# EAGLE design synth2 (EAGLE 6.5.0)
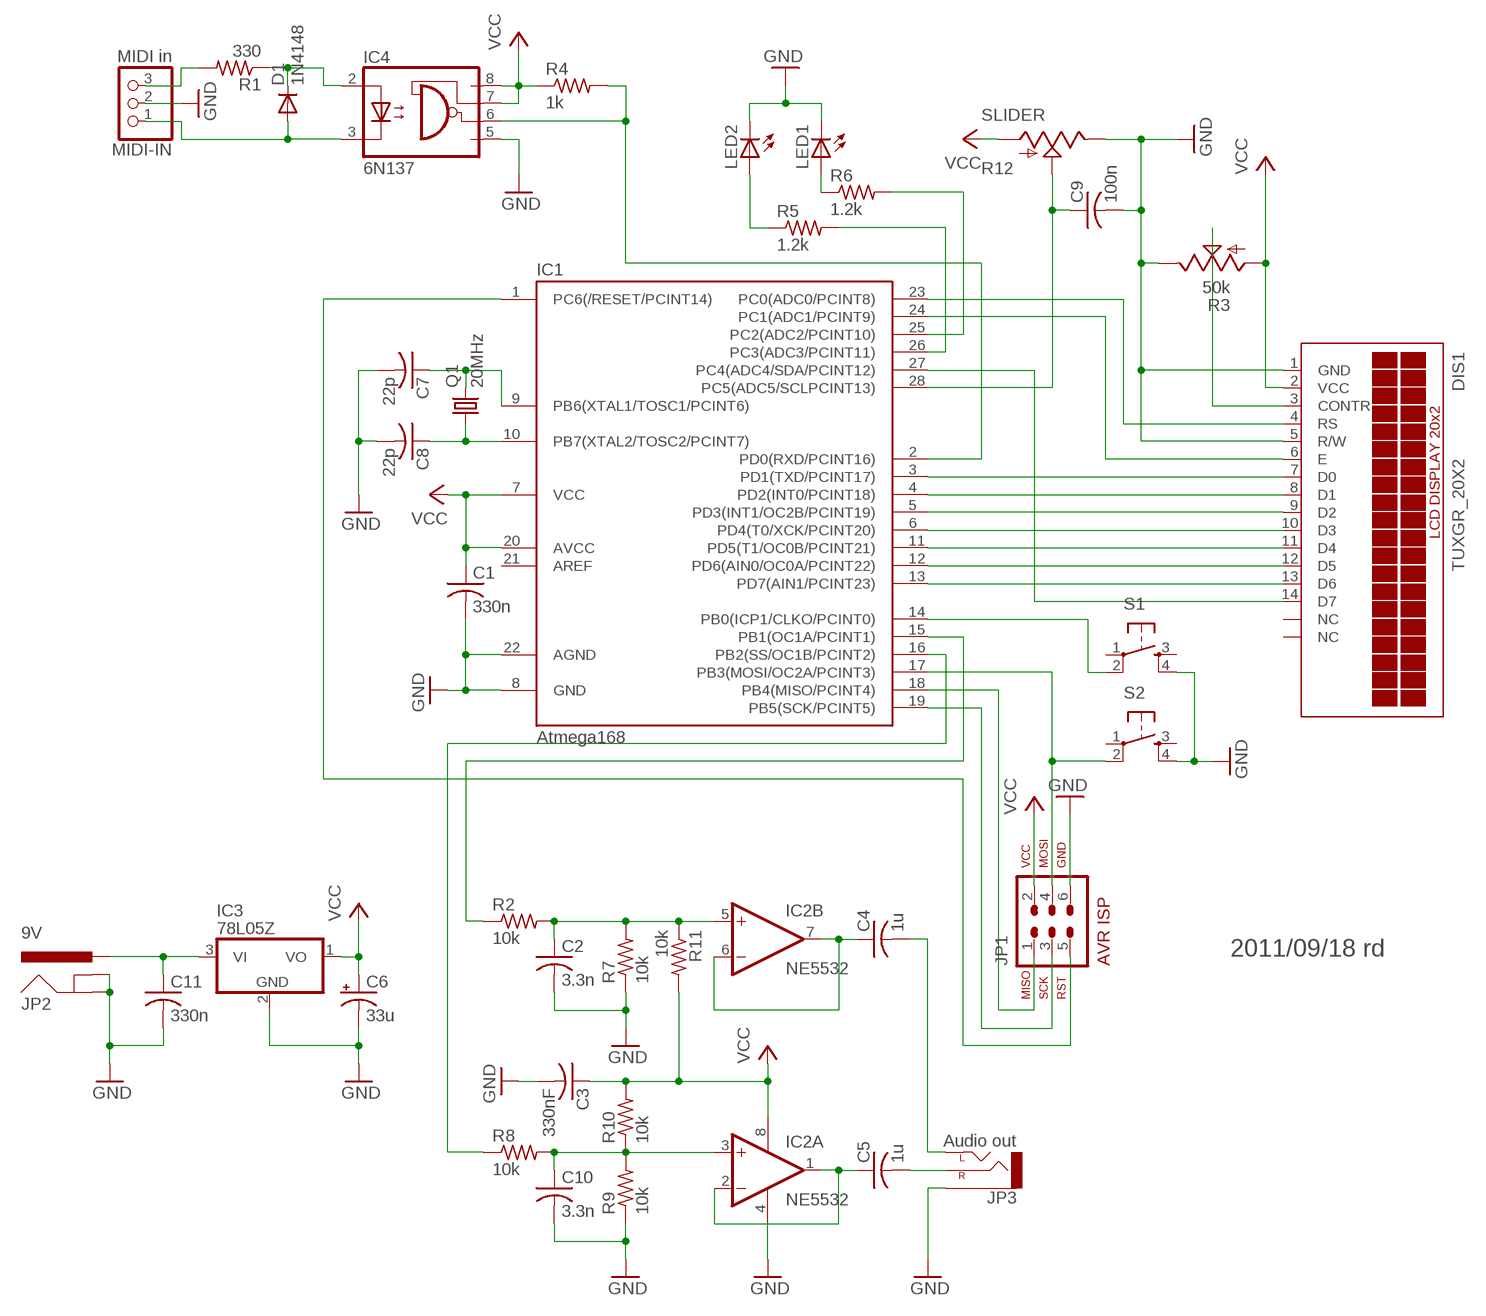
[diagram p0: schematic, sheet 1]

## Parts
C1  330n  C-USC0805  [C0805]
C2  3.3n  C-USC0805  [C0805]
C3  330nF  C-USC0805  [C0805]
C4  1u  C-USC0805  [C0805]
C5  1u  C-USC0805  [C0805]
C6  33u  CPOL-USCT7343  [CT7343]
C7  22p  C-USC0805  [C0805]
C8  22p  C-USC0805  [C0805]
C9  100n  C-USC0805  [C0805]
C10  3.3n  C-USC0805  [C0805]
C11  330n  C-USC0805  [C0805]
D1  1N4148  DIODE-SOD80C  [SOD80C]
DIS1  TUXGR_20X2  [TUXGR_20X2]
IC1  Atmega168  MEGA48/88/168-PU  [DIL28-3]
IC2  NE5532  TLC27L2ACP  [DIL08]
IC3  78L05Z  [TO92]
IC4  6N137  [DIL08]
JP1  AVR-ISP-6VERT  [AVR-ISP-6]
JP2  9V  POWER_JACKPTH  [POWER_JACK_PTH]
JP3  Audio out  AUDIO-JACKPTH  [AUDIO-JACK]
LED1  LED5MM  [LED5MM]
LED2  LED5MM  [LED5MM]
MIDI-IN  MIDI in  PINHD-1X3M  [1X03M]
Q1  20MHz  CRYSTALHC49U70  [HC49U70]
R1  330  R-US_R0805  [R0805]
R2  10k  R-US_R0805  [R0805]
R3  50k  TRIM_US-CA6V  [CA6V]
R4  1k  R-US_R0805  [R0805]
R5  1.2k  R-US_R0805  [R0805]
R6  1.2k  R-US_R0805  [R0805]
R7  10k  R-US_R0805  [R0805]
R8  10k  R-US_R0805  [R0805]
R9  10k  R-US_R0805  [R0805]
R10  10k  R-US_R0805  [R0805]
R11  10k  R-US_R0805  [R0805]
R12  SLIDER  [SLIDER]
S1  TAC_SWITCHPTH  [TACTILE-PTH]
S2  TAC_SWITCHPTH  [TACTILE-PTH]

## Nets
GND [Power]: C1.2 C2.2 C3.2 C6.- C7.2 C8.2 C9.2 C10.2 C11.2 DIS1.1(GND) DIS1.5(R/W) IC1.8(GND) IC1.22(AGND) IC2.4(C:GND) IC3.2(GND) IC4.5(GND) JP1.6 JP2.GND JP2.GNDBREAK JP3.SLEEVE LED1.K(C) LED2.K(C) MIDI-IN.2 R3.E R7.1 R9.1 R12.1(E) S1.4 S2.4
N$1: IC1.1(PC6(/RESET/PCINT14)) JP1.5
N$2: DIS1.4(RS) IC1.23(PC0(ADC0/PCINT8))
N$3: DIS1.6(E) IC1.24(PC1(ADC1/PCINT9))
N$4: D1.C IC4.2(A) R1.1
N$5: D1.A IC4.3(C) MIDI-IN.1
N$6: MIDI-IN.3 R1.2
N$7: DIS1.7(D0) IC1.3(PD1(TXD/PCINT17))
N$8: IC1.17(PB3(MOSI/OC2A/PCINT3)) JP1.4 S2.2
N$9: IC1.18(PB4(MISO/PCINT4)) JP1.1
N$10: IC1.19(PB5(SCK/PCINT5)) JP1.3
N$11: C2.1 IC2.5(B:+IN) R2.2 R7.2 R11.1
N$12 [Power]: DIS1.3(CONTR) R3.S
N$13: C4.1 IC2.6(B:-IN) IC2.7(B:OUT)
N$14: IC1.16(PB2(SS/OC1B/PCINT2)) R8.1
N$15: C4.2 JP3.TIP(LEFT)
N$16: C10.1 IC2.3(A:+IN) R8.2 R9.2 R10.1
N$17: C8.1 IC1.10(PB7(XTAL2/TOSC2/PCINT7)) Q1.1
N$18: C7.1 IC1.9(PB6(XTAL1/TOSC1/PCINT6)) Q1.2
N$19: IC1.15(PB1(OC1A/PCINT1)) R2.1
N$20: C9.1 IC1.28(PC5(ADC5/SCLPCINT13)) R12.2A(S)
N$21: IC1.14(PB0(ICP1/CLKO/PCINT0)) S1.2
N$22: DIS1.11(D4) IC1.11(PD5(T1/OC0B/PCINT21))
N$23: DIS1.8(D1) IC1.4(PD2(INT0/PCINT18))
N$24: DIS1.9(D2) IC1.5(PD3(INT1/OC2B/PCINT19))
N$25: DIS1.10(D3) IC1.6(PD4(T0/XCK/PCINT20))
N$26: DIS1.12(D5) IC1.12(PD6(AIN0/OC0A/PCINT22))
N$27: DIS1.13(D6) IC1.13(PD7(AIN1/PCINT23))
N$28: IC1.2(PD0(RXD/PCINT16)) IC4.6(VO) R4.2
N$29: IC1.25(PC2(ADC2/PCINT10)) R6.2
N$30: LED2.A R5.1
N$31: LED1.A R6.1
N$32: IC1.26(PC3(ADC3/PCINT11)) R5.2
N$33: DIS1.14(D7) IC1.27(PC4(ADC4/SDA/PCINT12))
N$35: C5.1 IC2.1(A:OUT) IC2.2(A:-IN)
N$36: C5.2 JP3.RING(RIGHT)
N$37: C11.1 IC3.3(VI) JP2.PWR
VCC [Power]: C1.1 C3.1 C6.+ DIS1.2(VCC) IC1.7(VCC) IC1.20(AVCC) IC2.8(C:VDD) IC3.1(VO) IC4.7(VE) IC4.8(VCC) JP1.2 R3.A R4.1 R10.2 R11.2 R12.3(A)
Unconnected: IC1.21(AREF) S1.1 S1.3 S2.1 S2.3

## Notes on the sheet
- 2011/09/18 rd

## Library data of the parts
C1-C5 C7-C11 = rcl:C-US: CAPACITOR, American symbol
C6 = rcl:CPOL-US: POLARIZED CAPACITOR, American symbol
D1 = diode:DIODE-: DIODE
DIS1 = display-lcd:TUXGR_20X2: Tuxgraphics LCD display 20x2 characters reflective, without background light Source: tuxgr_20x2.pdf; OC_FARNELL: unknown; OC_NEWARK: unknown
IC1 = avr-7:MEGA48/88/168-PU
IC2 = linear:TLC27L*: LinCMOS(TM) PRECISION DUAL OPERATIONAL AMPLIFIERS Source: http://focus.ti.com/lit/ds/symlink/tlc27l2.pdf
IC3 = linear:78*: Positive VOLTAGE REGULATOR Source: http://cache.national.com/ds/LM/LM78L05.pdf http://www.fairchildsemi.com/ds/LM/LM7805.pdf
IC4 = optocoupler:6N137: MOTOROLA OPTO COUPLER; MPN: 6N137; OC_FARNELL: 1328376; OC_NEWARK: 52M1895
JP1 = avr-7:AVR-ISP-6: AVR ISP-6 Serial Programming Header
JP2 = SparkFun-Connectors:POWER_JACK: Power Jack This is the standard 5.5mm barrel jack for power. The PTH is the most common, proven, reliable, footprint. The Slot footprint only works if the mill layer is transmitted to the PCB fab house so be warned. Mating wall wart : TOL-00298 (and others); PROD_ID: CONN-08197
JP3 = SparkFun:AUDIO-JACK: 3.5mm Audio Jack Simple 3.5mm common PCB mount audio jack. SKU: PRT-08032
LED1 LED2 = led:LED: LED
MIDI-IN = pinhead:PINHD-1X3: PIN HEADER
Q1 = crystal:CRYSTAL: CRYSTAL; OC_FARNELL: unknown; OC_NEWARK: unknown
R1 R2 R4-R11 = rcl:R-US_: RESISTOR, American symbol
R3 = pot:TRIM_US-: POTENTIOMETER
R12 = SparkFun:SLIDER
S1 S2 = SparkFun:TAC_SWITCH: Momentary Switch Button commonly used for reset or general input. Spark Fun Electronics SKU : COM-00097

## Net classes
0 default: width 0.254 mm
1 Power: width 0.508 mm

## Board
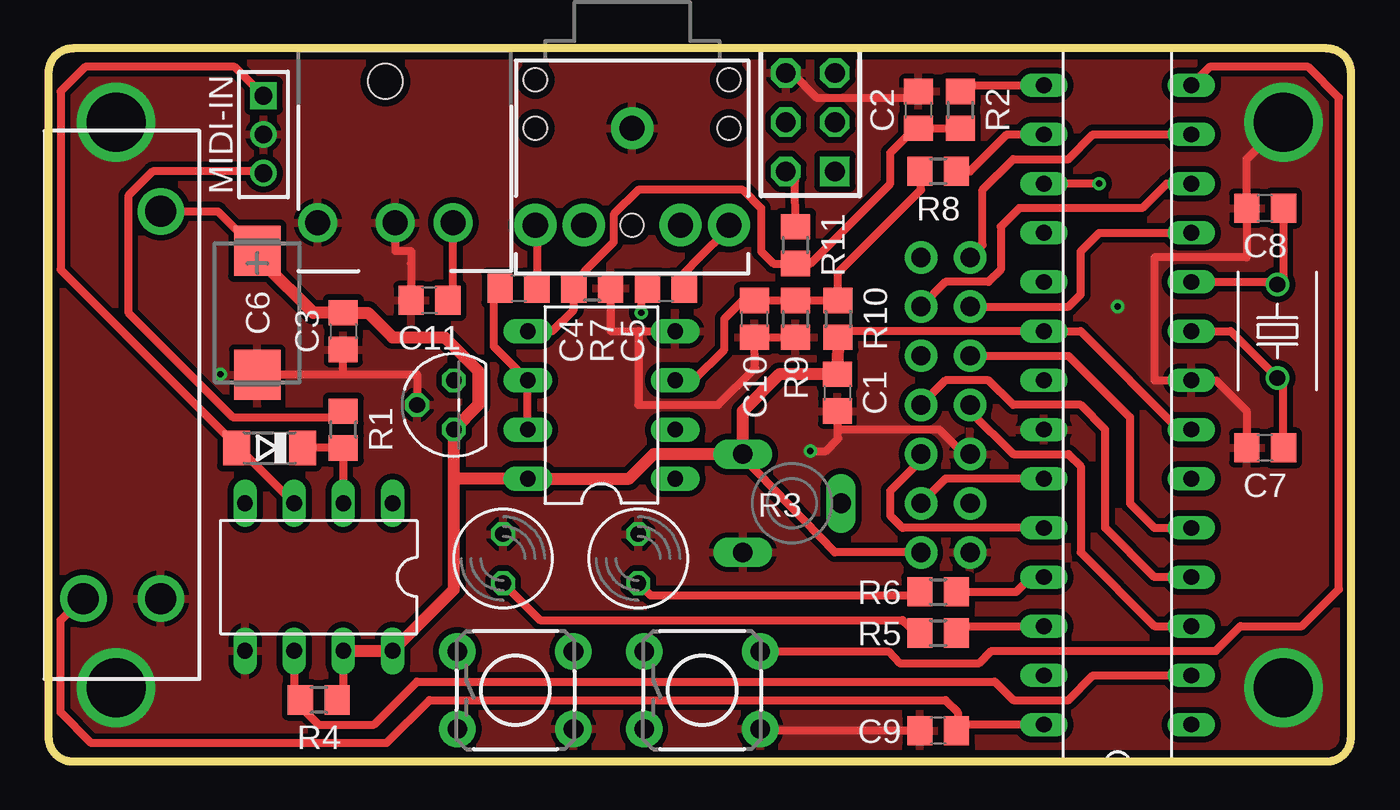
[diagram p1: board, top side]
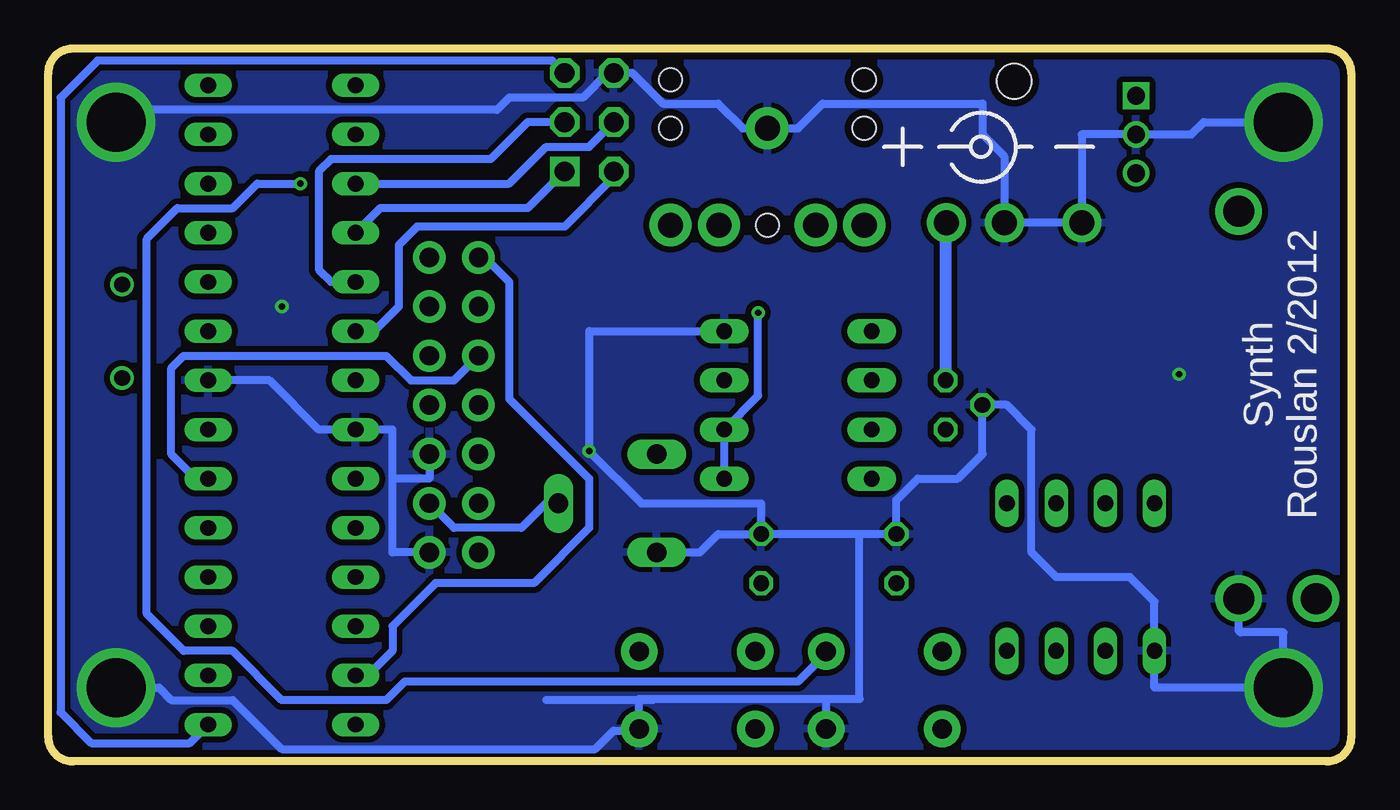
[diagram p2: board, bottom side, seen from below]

Size 67.31 x 36.83 mm. Coordinates in mm from the lower left corner, seen from the top.
Outline: 1.27,0 66.04,0 arc90 67.31,1.27 67.31,35.56 arc90 66.04,36.83 1.27,36.83 arc90 0,35.56 0,1.27 arc90 1.27,0
Copper layers (1*16): Top 0.0356mm / dielectric 1.5011mm / Bottom 0.0356mm
Design rules "LaenPCBOrder *": minimum track width 6mil, minimum drill 13mil, track to track 6mil, track to pad 6mil, pad to pad 6mil, via to via 6mil, smd to smd 6mil, copper to edge 15mil, drill to drill 6mil, minimum pad ring 7mil, minimum via ring 7mil, stop-mask expansion 3mil, vias tented up to drill 15mil, thermal gap 10mil

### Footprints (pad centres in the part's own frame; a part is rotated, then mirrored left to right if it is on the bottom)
C0805 = smd 1.3 x 1.5: 1 -0.95,0; 2 0.95,0
CT7343 = smd 2.6 x 2.4: + -3.2,0; - 3.2,0
SOD80C = smd 1.4 x 1.8: A 1.7,0; C -1.7,0
TUXGR_20X2 = drill 1 pad 1.676: 1 1.27,-7.62; 2 -1.27,-7.62; 3 1.27,-5.08; 4 -1.27,-5.08; 5 1.27,-2.54; 6 -1.27,-2.54; 7 1.27,0; 8 -1.27,0; 9 1.27,2.54; 10 -1.27,2.54; 11 1.27,5.08; 12 -1.27,5.08; 13 1.27,7.62; 14 -1.27,7.62
DIL28-3 = drill 0.813 long: 1 -16.51,-3.81; 2 -13.97,-3.81; 3 -11.43,-3.81; 4 -8.89,-3.81; 5 -6.35,-3.81; 6 -3.81,-3.81; 7 -1.27,-3.81; 8 1.27,-3.81; 9 3.81,-3.81; 10 6.35,-3.81; 11 8.89,-3.81; 12 11.43,-3.81; 13 13.97,-3.81; 14 16.51,-3.81; 15 16.51,3.81; 16 13.97,3.81; 17 11.43,3.81; 18 8.89,3.81; 19 6.35,3.81; 20 3.81,3.81; 21 1.27,3.81; 22 -1.27,3.81; 23 -3.81,3.81; 24 -6.35,3.81; 25 -8.89,3.81; 26 -11.43,3.81; 27 -13.97,3.81; 28 -16.51,3.81
DIL08 = drill 0.813 pad 1.27 long: 1 -3.81,-3.81; 2 -1.27,-3.81; 3 1.27,-3.81; 4 3.81,-3.81; 5 3.81,3.81; 6 1.27,3.81; 7 -1.27,3.81; 8 -3.81,3.81
TO92 = drill 0.813 octagon: 1 -1.27,0; 2 0,1.905; 3 1.27,0
DIL08' = drill 0.813 long: 1 -3.81,-3.81; 2 -1.27,-3.81; 3 1.27,-3.81; 4 3.81,-3.81; 5 3.81,3.81; 6 1.27,3.81; 7 -1.27,3.81; 8 -3.81,3.81
AVR-ISP-6 = drill 1.016 square: 1 -2.54,-1.27 | drill 1.016 octagon: 2 -2.54,1.27; 3 0,-1.27; 4 0,1.27; 5 2.54,-1.27; 6 2.54,1.27
POWER_JACK_PTH = drill 1.3 pad 2: GND 4.5,9; GNDBREAK 0.5,9; PWR -2.5,9 | hole 1.8: 1,1.7
AUDIO-JACK = drill 1.3 pad 2.184: RING 5,5; RSH 5,2.5; SLEEVE 0,0; TIP 5,-5; TSH 5,-2.5 | hole 1.2: 0,5; -2.5,5; -2.5,-5; 0,-5; 5,0
LED5MM = drill 0.813 octagon: A -1.27,0; K 1.27,0
1X03M = drill 0.914 square: 1 -2,0 | drill 0.914: 2 0,0; 3 2,0
HC49U70 = drill 0.813: 1 -2.413,0; 2 2.413,0
R0805 = smd 1.3 x 1.5: 1 -0.95,0; 2 0.95,0
CA6V = drill 1.016 long: A -2.54,-2.54; E 2.54,-2.54; S 0,2.54
SLIDER = drill 1.6 pad 2: 1 10,2; 2A 10,-2; 3 -10,2
TACTILE-PTH = drill 1.016 pad 1.88: 1 -3,2; 2 3,2; 3 -3,-2; 4 3,-2

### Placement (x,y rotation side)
C1  40.77,19.05 270 top
C2  44.96,33.65 90 top
C3  15.24,22.23 270 top
C4  24.29,24.45 0 top
C5  31.91,24.45 0 top
C6  10.79,23.18 270 top
C7  62.87,16.19 180 top
C8  62.87,28.57 180 top
C9  45.97,1.59 180 top
C10  36.48,22.86 270 top
C11  19.68,23.81 180 top
D1  11.43,16.19 180 top
DIS1  46.35,18.41 0 top
IC1  55.24,18.41 90 top
IC2  28.57,18.41 90 top
IC3  20.96,18.41 90 top
IC4  6N137  [DIL08']  13.97,9.53 180 top
JP1  39.37,33.02 90 top
JP2  18.41,36.83 180 top
JP3  30.16,32.7 270 top
LED1  30.48,10.48 90 top
LED2  23.5,10.48 90 top
MIDI-IN  11.11,32.38 270 top
Q1  63.5,22.23 270 top
R1  15.24,17.14 90 top
R2  47.12,33.65 270 top
R3  38.42,13.33 270 top
R4  13.97,3.17 180 top
R5  45.97,6.64 0 top
R6  45.97,8.76 0 top
R7  28.1,24.45 180 top
R8  45.97,30.48 180 top
R9  38.61,22.86 90 top
R10  40.8,22.86 270 top
R11  38.61,26.67 90 top
R12  3.81,18.41 270 top
S1  33.78,3.68 0 top
S2  24.13,3.68 0 top

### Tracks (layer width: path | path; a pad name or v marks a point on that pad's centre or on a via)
GND  (via drill 0.33, 3.05)
  Top 0.406: C7.2 61.91,18.09 60.32,19.69 IC1.8 57.15,19.69 57.15,26.03 61.91,26.03 C8.2 61.91,31.12 v63.82,33.02 | DIS1.5 47.31,15.87 46.04,17.14 40.8,17.14 | 40.8,17.14 C1.2 | R9.1 C10.2 36.51,20.32 34.61,18.41 30.48,18.41 30.48,22.23 | 30.48,22.23 29.05,22.23 R7.1 | 30.48,22.23 IC2.4 | C9.2 37.2,1.59 S1.4 | C6.- 10.82,20 15.24,20 | 15.24,20 C3.2 | 15.24,20 19.05,20 IC3.2 | JP1.6 38.42,35.56 39.69,34.29 44.77,34.29 C2.2 | v39.37,16.03 40.16,16.03 40.8,16.67 40.8,17.14 | JP2.GNDBREAK 17.91,26.38 18.73,26.38 18.73,25.72 C11.2
  Bottom 0.406: v3.49,33.02 7.62,33.02 8.26,32.38 MIDI-IN.2 13.92,32.38 JP2.GND JP2.GNDBREAK 17.91,31.25 19.05,32.38 19.05,33.97 27.3,33.97 28.57,32.7 JP3.SLEEVE 31.43,32.7 32.7,33.97 35.56,33.97 37.15,35.56 JP1.6 38.42,35.56 39.69,34.29 43.5,34.29 44.13,33.65 63.18,33.65 v63.82,33.02 | 25.4,11.75 LED2.K 23.5,13.49 22.38,14.6 20.32,14.6 19.05,15.87 IC3.2 17.78,18.41 16.51,17.14 16.51,10.79 15.24,9.53 11.43,9.53 10.16,8.26 IC4.5 10.16,3.81 v3.49,3.81 3.49,6.67 5.71,6.67 5.81,6.76 R12.1 | 25.4,11.75 LED1.K | 25.4,11.75 25.4,3.22 27.13,3.22 | 27.13,3.22 36.81,3.22 | 36.81,3.22 S1.4 36.88,1.59 38.1,1.59 39.05,0.63 55.24,0.63 57.78,3.17 60.96,3.17 61.59,3.81 v63.82,3.81 | 27.13,3.22 S2.4 | 36.81,3.22 36.07,3.17 41.59,3.17 | 49.53,14.6 47.62,14.6 DIS1.5 | 49.53,14.6 49.53,17.14 IC1.22 53.34,17.14 55.88,19.69 IC1.8 | DIS1.1 49.53,10.79 49.53,14.6 | R3.E 33.65,10.79 32.7,11.75 LED1.K | IC2.4 39.37,22.23 v39.37,16.03 36.67,13.33 30.48,13.33 LED1.K
  other vias: 8.89,20 8.89,20 55.24,23.49
  pour Bottom (isolate 0.305): -1.27,37.46 -1.27,-0.64 68.58,-0.64 68.58,37.46
  pour Top (isolate 0.305): -2.54,38.73 -2.54,-1.91 69.85,-1.91 69.85,38.73
N$1
  Bottom 0.406: JP1.5 41.27,36.2 64.77,36.2 66.67,34.29 66.67,2.54 65.09,0.95 60.01,0.95 IC1.1
N$2
  Top 0.406: IC1.23 46.35,14.6 DIS1.4
N$3
  Top 0.406: IC1.24 44.13,12.06 43.5,12.7 43.5,13.97 45.08,15.56 DIS1.6
N$4
  Top 0.406: IC4.2 R1.1 D1.C
N$5
  Top 0.406: IC4.3 9.84,16.19 D1.A 9.73,16.3 0.64,25.4 0.64,34.61 1.9,35.88 9.62,35.88 MIDI-IN.1
N$6
  Top 0.406: MIDI-IN.3 11.02,30.48 5.4,30.48 4.13,29.21 4.13,23.18 9.53,17.78 14.93,17.78 R1.2
N$7
  Top 0.406: DIS1.7 47.62,18.1 49.85,15.87 52.7,15.87 53.34,15.24 53.34,10.79 57.15,6.98 IC1.3
N$8  (via drill 0.33)
  Top 0.406: v54.29,29.84 IC1.17
  Bottom 0.406: IC1.17 43.5,29.84 41.59,31.75 39.37,31.75 JP1.4 | S2.2 27.13,5.57 28.57,4.13 48.89,4.13 49.85,3.17 55.24,3.17 57.78,5.71 60.32,5.71 62.23,7.62 62.23,26.99 60.64,28.57 57.78,28.57 56.51,29.84 v54.29,29.84
N$9
  Bottom 0.406: JP1.1 42.54,28.57 50.16,28.57 IC1.18
N$10
  Bottom 0.406: JP1.3 42.54,33.02 44.45,31.11 52.7,31.11 53.34,30.48 53.34,25.4 52.7,24.77 IC1.19
N$11
  Top 0.406: IC2.5 26.04,22.23 27.15,23.34 R7.2 27.78,25.4 29.21,26.83 29.21,28.26 30.48,29.53 35.88,29.53 36.83,28.57 36.83,26.35 37.46,25.72 38.41,25.72 R11.1 39.37,25.72 43.5,29.84 43.5,31.43 44.77,32.7 C2.1 R2.2
N$12
  Bottom 0.406: DIS1.3 46.35,12.06 42.86,12.06 41.59,13.33 R3.S
N$13
  Top 0.406: IC2.7 IC2.6 23.02,21.43 23.02,23.02 23.02,24.13 C4.1
N$14
  Top 0.406: R8.1 47.62,30.48 49.53,32.38 IC1.16
N$15
  Top 0.406: JP3.TIP 25.24,27.47 C4.2
N$16
  Top 0.406: IC2.3 33.34,19.69 34.92,21.27 34.92,22.86 35.88,23.81 36.51,23.81 C10.1 R9.2 R10.1 40.8,25.24 45.08,29.53 45.08,30.48 R8.2
  Bottom 0.406: IC2.3 33.34,19.69
N$17
  Top 0.406: C8.1 63.81,24.95 Q1.1 63.37,24.77 IC1.10
N$18
  Top 0.406: C7.1 63.81,19.5 Q1.2 61.09,22.23 IC1.9
N$19
  Top 0.406: R2.1 47.62,34.92 IC1.15
N$20
  Top 0.406: R12.2A 1.81,8.48 0.64,7.3 0.64,2.54 2.22,0.95 17.46,0.95 19.68,3.17 46.35,3.17 46.99,2.54 46.99,1.59 C9.1 47.3,1.9 IC1.28
N$21
  Top 0.406: S1.2 43.4,5.68 43.97,5.08 48.1,5.08 48.74,5.71 60.32,5.71 61.59,6.98 64.77,6.98 66.67,8.89 66.67,34.29 65.09,35.88 60.01,35.88 IC1.14
N$22
  Top 0.406: DIS1.11 52.7,23.49 53.34,24.13 53.34,26.35 54.29,27.3 IC1.11
N$23
  Top 0.406: IC1.4 57.15,9.53 54.61,12.06 54.61,17.14 53.34,18.41 49.85,18.41 48.58,19.69 46.35,19.69 DIS1.8
N$24
  Top 0.406: DIS1.9 52.7,20.95 55.88,17.78 55.88,13.33 57.15,12.06 IC1.5
N$25
  Bottom 0.406: IC1.6 59.69,14.6 60.96,15.87 60.96,20.32 60.32,20.95 49.85,20.95 48.58,19.69 46.35,19.69 DIS1.10
N$26
  Top 0.406: IC1.12 57.78,29.84 56.51,28.57 50.16,28.57 49.21,27.62 49.21,25.4 48.58,24.77 46.35,24.77 DIS1.12
N$27
  Top 0.406: DIS1.13 48.26,26.67 48.26,29.53 49.85,31.11 52.7,31.11 53.97,32.38 IC1.13
N$28
  Top 0.406: IC4.6 12.7,3.49 R4.2 13.02,2.85 13.97,1.9 16.83,1.9 19.05,4.13 48.89,4.13 49.85,3.17 52.7,3.17 53.97,4.44 IC1.2
N$29
  Top 0.406: R6.2 50.01,8.76 50.8,9.53 IC1.25
N$30
  Top 0.406: LED2.A 25.4,7.3 44.13,7.3 44.45,6.98 R5.1
N$31
  Top 0.406: LED1.A 31.11,8.57 44.77,8.57 45.08,8.26 R6.1
N$32
  Top 0.406: R5.2 47.15,6.98 IC1.26
N$33
  Bottom 0.406: DIS1.14 44.77,26.03 43.5,24.77 43.5,18.73 39.37,14.6 39.37,12.06 42.23,9.21 47.31,9.21 49.53,6.98 49.53,5.71 50.8,4.44 IC1.27
N$35  (via drill 0.33)
  Top 0.406: v30.64,23.18 30.64,24.13 C5.1
  Bottom 0.406: v30.64,23.18 30.64,18.89 IC2.2 IC2.1
N$36
  Top 0.406: C5.2 32.86,25.24 33.65,26.03 35.08,27.46 JP3.RING
N$37
  Top 0.406: C11.1 20.91,24.09 JP2.PWR
  Bottom 0.61: JP2.PWR 20.96,27.15 IC3.3
VCC
  Top 0.406: IC4.7 15.24,3.49 R4.1 | R10.2 40.8,22.23 IC1.20 53.34,22.23 58.42,17.14 IC1.7 | DIS1.2 40.64,10.79 35.88,15.72 R3.A | R11.2 38.58,30 JP1.2 | R12.3 8.76,28.41 C6.+
  Top 0.61: IC4.7 IC4.8 20.96,8.89 20.96,14.6 | 20.96,14.6 IC3.1 22.23,18.41 22.23,20.16 20.48,21.91 17.78,21.91 16.51,23.17 C3.1 13.68,23.17 11.11,25.72 10.79,26.03 C6.+ | 20.96,14.6 IC2.8 30,14.6 31.27,15.87 R3.A 35.88,18.09 37.78,20 C1.1 40.8,22.23
  Bottom 0.406: JP1.2 38.1,30.16 40.64,27.62 48.26,27.62 49.21,26.67 49.21,23.49 50.48,22.23 IC1.20

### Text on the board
bNames: Synth / Rouslan 2/2012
